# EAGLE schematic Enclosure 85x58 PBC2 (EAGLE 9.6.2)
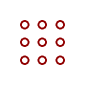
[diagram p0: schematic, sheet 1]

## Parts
U$1  PROTO-28X18-S1A  [PROTO-28X18-S1A]

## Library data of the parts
U$1 = digitalconcepts:PROTO-28X18-S1A: 28 x 18 Prototyping board to fit an 85 x 58 enclosure, with external connector cut-outs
